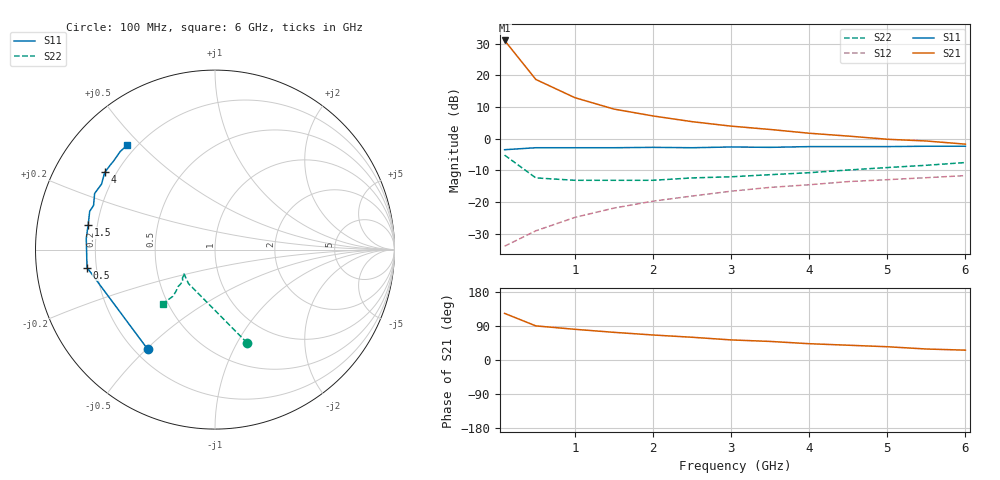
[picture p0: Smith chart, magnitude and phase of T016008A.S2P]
!AT-00600
!S-PARAMETERS at Vce=8V  Ic=35mA.  LAST UPDATED 07-21-92
# ghz s ma r 50
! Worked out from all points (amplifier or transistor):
!   13 points, 100 MHz to 6 GHz, reference 50 ohm
!   highest |S21| = 31.1 dB at 100 MHz (marker M1)
!   |S21| within 3 dB of that: start of sweep to 197.3 MHz
!   unconditionally stable (mu >= 1): 763 MHz to 5.034 GHz
!   at 1 GHz: K = 1.09, MAG = 17.1 dB, |S12| = -24.9 dB
!   at 3 GHz: K = 1.07, MAG = 8.7 dB, |S12| = -16.6 dB
!   at 6 GHz: K = 0.95, MSG = 5.0 dB, |S12| = -11.7 dB
!   S11 on the Smith chart (normalised r, x): 100 MHz: 0.25, -0.51; 500 MHz: 0.16, -0.07; 1.5 GHz: 0.16, +0.09; 4 GHz: 0.16, +0.31; 6 GHz: 0.17, +0.46
0.1  0.67 -124.0  35.75 123.0  0.02 47.0  0.55 -71.0
0.5  0.72 -172.0  8.64 90.0  0.035 53.0  0.24 -128.0
1  0.72 175.0  4.45 81.0  0.057 65.0  0.22 -141.0
1.5  0.72 169.0  2.94 73.0  0.08 69.0  0.22 -143.0
2  0.73 163.0  2.29 66.0  0.103 71.0  0.22 -141.0
2.5  0.72 160.0  1.86 60.0  0.124 72.0  0.24 -139.0
3  0.74 155.0  1.58 53.0  0.148 70.0  0.25 -136.0
3.5  0.73 150.0  1.4 49.0  0.17 71.0  0.27 -135.0
4  0.75 145.0  1.22 43.0  0.187 69.0  0.29 -135.0
4.5  0.75 141.0  1.1 39.0  0.21 69.0  0.32 -133.0
5  0.75 139.0  0.98 35.0  0.225 67.0  0.35 -132.0
5.5  0.76 134.0  0.92 29.0  0.242 67.0  0.38 -133.0
6  0.76 130.0  0.82 26.0  0.261 66.0  0.42 -134.0
